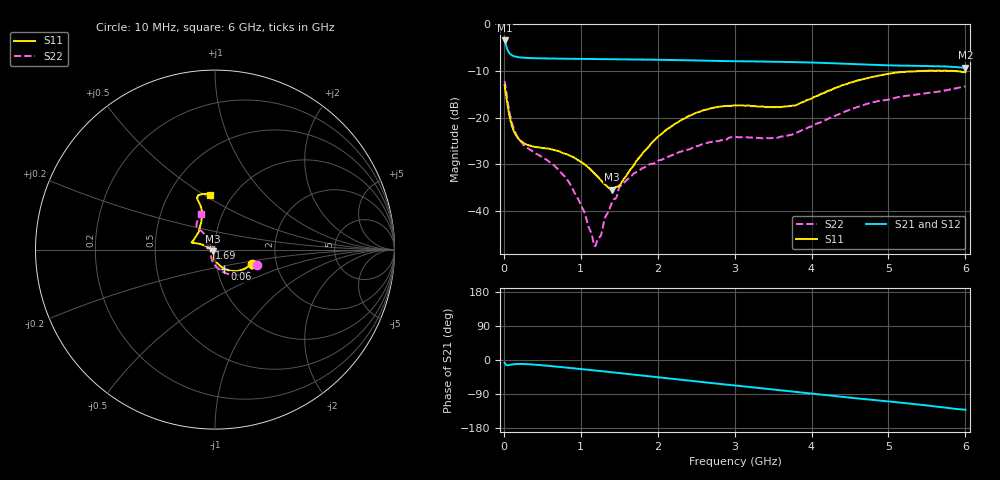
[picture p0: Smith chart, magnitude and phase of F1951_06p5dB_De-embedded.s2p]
! Integrated Device Technology
! Corporate Headquarters
! 6024 Silver Creek Valley Road
! San Jose, CA 95138  USA
! Phone:  1-408-284-8200
! Toll Free:  1-800-223-1366
! Webpage:  http://www.idt.com/
! Timing and RF Division
! 515 Groton Road, Suite 102
! Westford, MA 01886-6024
! Device:  F1951
! Description: 6-bit 0.5 dB Digital Step Attenuator
! Frequency:  100.0 -  4000.00 MHz
! Package:  4x4 mm Thin QFN Plastic Package: 24 pin
! Ports:  2 RF, 6 DC
!  Pin  1  = NC
!  Pin  2  = RF1  =  Port 1
!  Pin  3  = GND
!  Pin  4  = NC
!  Pin  5  = Serial Data Out (SDO)
!  Pin  6  = NC
!  Pin  7  = Reset Bar ( RSTb)
!  Pin  8  = Clock (CLK)
!  Pin  9  = Chip Select Bar (CSb)
!  Pin 10  = NC
!  Pin 11  = Serial Data In (SDI)
!  Pin 12  = NC
!  Pin 13  = NC
!  Pin 14  = VDD
!  Pin 15  = NC
!  Pin 16  = GND
!  Pin 17  = RF2  =  Port 2
!  Pin 18  = NC
!  Pin 19  = GND
!  Pin 20  = GND
!  Pin 21  = GND
!  Pin 22  = GND
!  Pin 23  = GND
!  Pin 24  = GND
! State:  13
! Atten State:  6.5 dB
! Voltage:  +3.30 Volts
! Current:  0.488 mA
! Data:  The device was measured on a F195X evaluation board which has
!  individual transmission lines to the RF pins.  Data was collected
!  de-embedded using a Automatic Fixture Removal [AFR] (Keysight Technologies).
!  The reference plane is the edge of the package pin.
! Misc:  Lot Code  1225BCA
!  Action Tracker AT0399
! Date Measured:  2018-09-13
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# GHz S dB R 50
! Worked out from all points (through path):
!   600 points, 10 MHz to 6 GHz, reference 50 ohm
!   highest |S21| = -3.50 dB at 10 MHz (marker M1); lowest = -9.3 dB at 6 GHz (marker M2)
!   group delay of S21, straight-line fit = 58.7 ps
!   lowest |S11| = -35.4 dB at 1.4 GHz (marker M3), VSWR 1.03, Z = 48.7 - j1.02 ohm
!   |S11| at or under -10 dB: start of sweep to 5.45 GHz; 5.767 GHz to 5.806 GHz (38.57 MHz wide, 0.666 % of centre); 5.842 GHz to end of sweep
!   |S22| runs from -47.5 to -12.2 dB; largest |S21 - S12| = 0.00061
!   S11 on the Smith chart (normalised r, x): 10 MHz: 1.50, -0.24; 60 MHz: 1.09, -0.23; 1.69 GHz: 0.94, +0.01; 6 GHz: 0.79, +0.53
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0.01  -13.08 -20.5  -3.50 -6.8  -3.50 -6.8  -12.18 -19.8
0.06  -18.49 -63.6  -5.90 -13.7  -5.90 -13.7  -17.65 -70.9
0.13  -22.85 -82.8  -6.85 -11.2  -6.85 -11.1  -22.35 -95.9
0.24  -25.22 -94.4  -7.17 -10.5  -7.17 -10.5  -25.50 -112.1
0.7  -27.10 -98.2  -7.38 -17.7  -7.38 -17.7  -30.97 -122.5
0.84  -27.99 -96.8  -7.41 -20.6  -7.41 -20.6  -33.64 -123.4
1.01  -29.53 -97.0  -7.45 -24.0  -7.45 -24.0  -39.01 -126.2
1.16  -31.64 -104.3  -7.47 -27.1  -7.47 -27.1  -46.32 -162.4
1.19  -32.14 -106.8  -7.47 -27.7  -7.47 -27.7  -47.48 174.1
1.25  -33.17 -113.0  -7.47 -29.0  -7.48 -29.0  -45.48 142.3
1.4  -35.38 -142.0  -7.50 -32.2  -7.50 -32.2  -38.38 109.3
1.52  -34.15 -171.7  -7.52 -34.7  -7.52 -34.7  -34.57 108.9
1.69  -30.16 166.5  -7.55 -38.5  -7.55 -38.5  -31.96 110.3
2.01  -23.99 158.8  -7.63 -45.6  -7.63 -45.6  -29.16 124.7
2.49  -19.02 161.6  -7.77 -56.2  -7.77 -56.2  -26.19 149.4
3.01  -17.35 163.3  -7.93 -67.3  -7.93 -67.3  -24.13 159.1
3.55  -17.73 145.6  -8.04 -79.0  -8.05 -79.0  -24.32 141.5
3.79  -17.39 130.7  -8.14 -84.3  -8.15 -84.2  -23.28 131.5
4.01  -15.79 119.2  -8.22 -89.1  -8.22 -89.1  -21.81 125.4
4.55  -12.31 108.2  -8.56 -100.4  -8.56 -100.4  -17.99 126.2
5.01  -10.62 109.3  -8.83 -109.5  -8.83 -109.5  -16.13 128.8
6  -10.29 95.0  -9.34 -131.3  -9.34 -131.3  -13.33 112.0
